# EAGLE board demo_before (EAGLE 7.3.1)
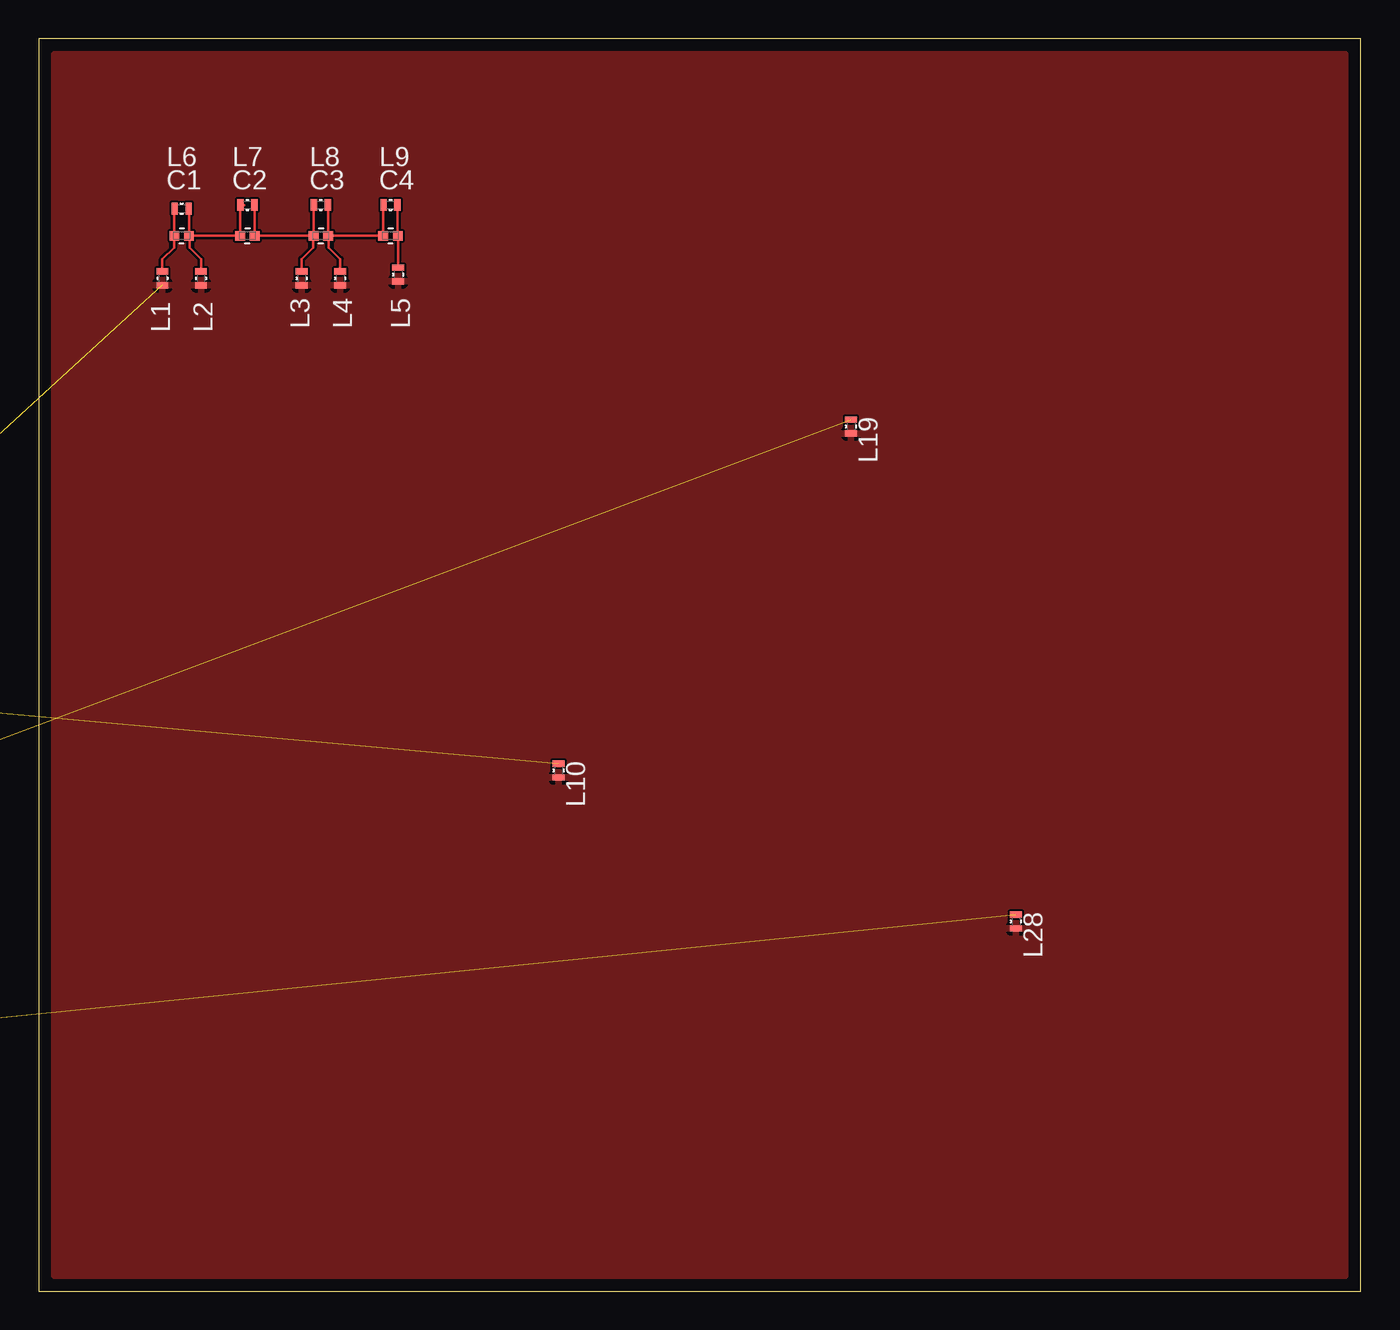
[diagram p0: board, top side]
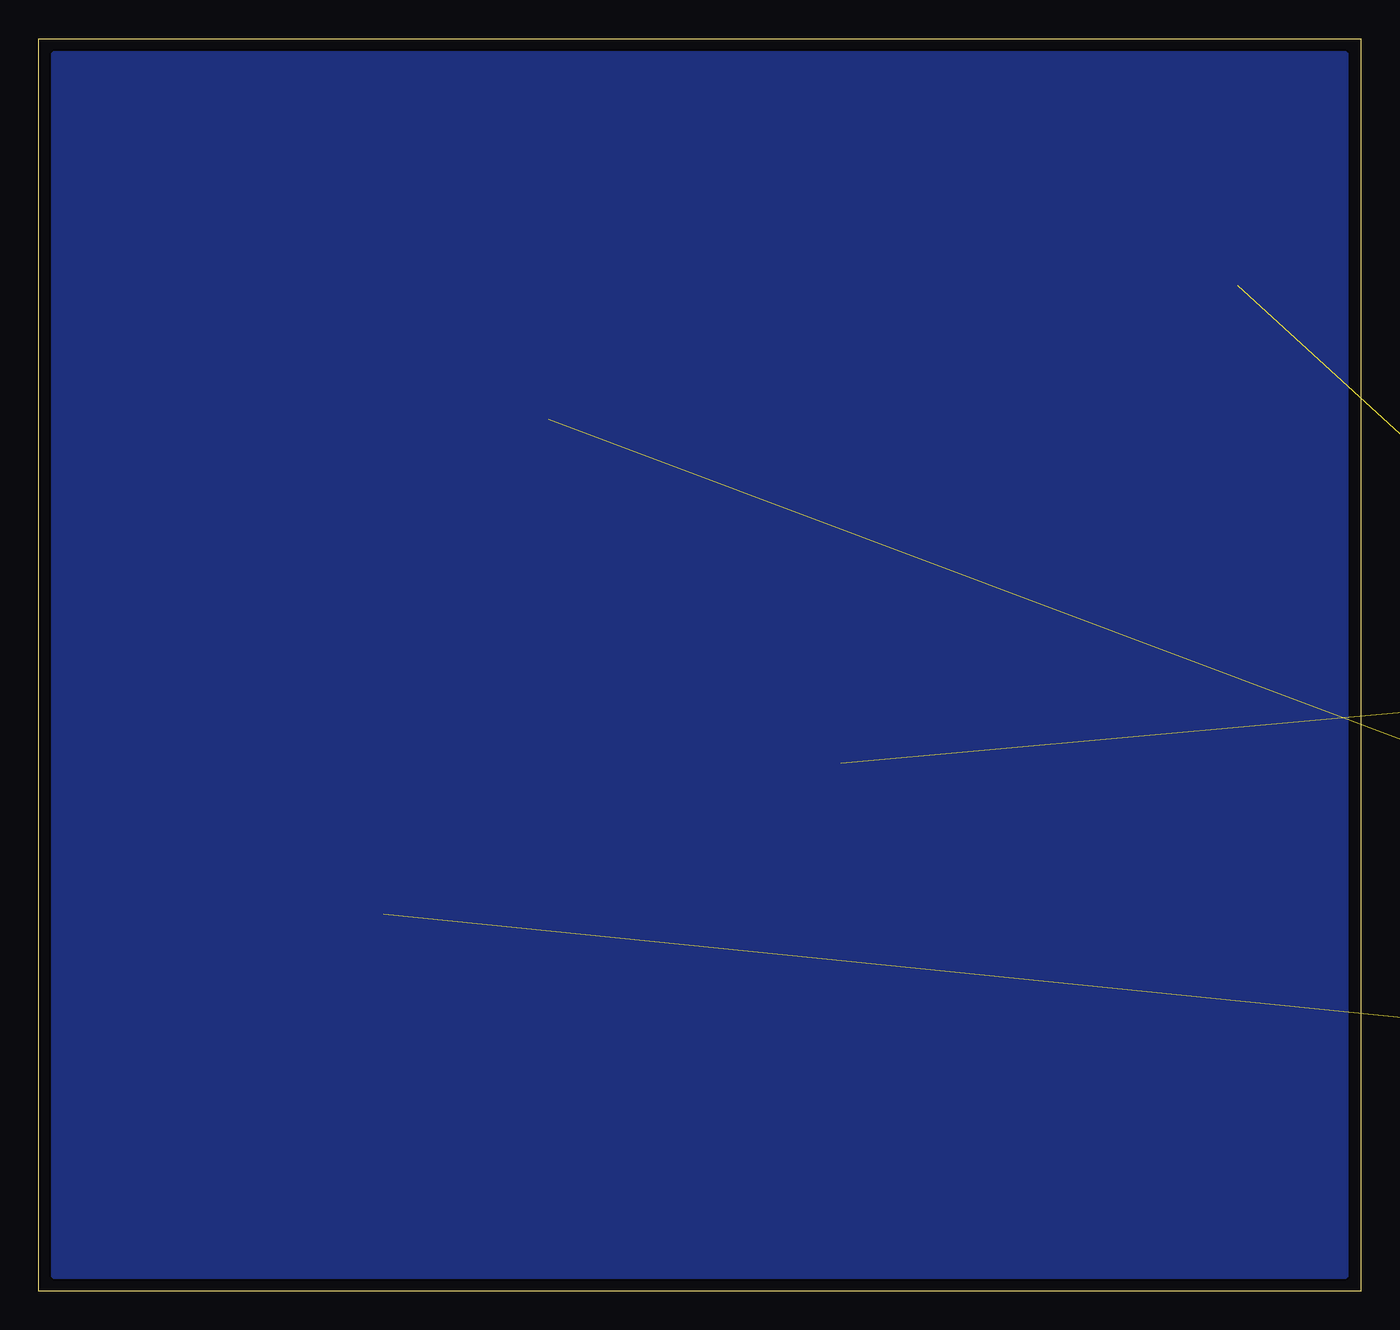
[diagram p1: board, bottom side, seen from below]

Size 85.5 x 81 mm. Coordinates in mm from the lower left corner, seen from the top.
Outline: 0,0 85.5,0 85.5,81 0,81 0,0
Copper layers (1*16): Top 0.0178mm / dielectric 59mil / Bottom 0.0178mm
Design rules "SSC-EAGLE-2Lyr_v1.0.0.3 *": minimum track width 6mil, minimum drill 14mil, track to track 6mil, track to pad 6mil, pad to pad 6mil, via to via 6mil, smd to smd 6mil, copper to edge 20mil, drill to drill 16mil, minimum pad ring 8mil, minimum via ring 8mil, stop-mask expansion 3mil, vias tented up to drill 0mil, thermal gap 10mil

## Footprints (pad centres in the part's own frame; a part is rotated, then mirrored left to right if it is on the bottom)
LTDB_PASSIVES_C0402 = smd 0.635 x 0.635: 1 -0.472,0; 2 0.472,0
LTDB_PASSIVES_R0402 = smd 0.406 x 0.762: 1 -0.447,0; 2 0.447,0

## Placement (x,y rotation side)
C1  [LTDB_PASSIVES_C0402]  9.25,68.25 0 top
C2  [LTDB_PASSIVES_C0402]  13.5,68.25 0 top
C3  [LTDB_PASSIVES_C0402]  18.25,68.25 0 top
C4  [LTDB_PASSIVES_C0402]  22.75,68.25 0 top
C5  [LTDB_PASSIVES_C0402]  not placed on the board
C6  [LTDB_PASSIVES_C0402]  not placed on the board
C7  [LTDB_PASSIVES_C0402]  not placed on the board
C8  [LTDB_PASSIVES_C0402]  not placed on the board
C9  [LTDB_PASSIVES_C0402]  not placed on the board
C10  [LTDB_PASSIVES_C0402]  not placed on the board
C11  [LTDB_PASSIVES_C0402]  not placed on the board
C12  [LTDB_PASSIVES_C0402]  not placed on the board
C13  [LTDB_PASSIVES_C0402]  not placed on the board
C14  [LTDB_PASSIVES_C0402]  not placed on the board
C15  [LTDB_PASSIVES_C0402]  not placed on the board
C16  [LTDB_PASSIVES_C0402]  not placed on the board
L1  [LTDB_PASSIVES_R0402]  8,65.5 270 top
L2  [LTDB_PASSIVES_R0402]  10.5,65.5 270 top
L3  [LTDB_PASSIVES_R0402]  17,65.5 270 top
L4  [LTDB_PASSIVES_R0402]  19.5,65.5 270 top
L5  [LTDB_PASSIVES_R0402]  23.25,65.75 270 top
L6  [LTDB_PASSIVES_R0402]  9.25,70 0 top
L7  [LTDB_PASSIVES_R0402]  13.5,70.25 0 top
L8  [LTDB_PASSIVES_R0402]  18.25,70.25 0 top
L9  [LTDB_PASSIVES_R0402]  22.75,70.25 0 top
L10  [LTDB_PASSIVES_R0402]  33.61,33.67 270 top
L11  [LTDB_PASSIVES_R0402]  not placed on the board
L12  [LTDB_PASSIVES_R0402]  not placed on the board
L13  [LTDB_PASSIVES_R0402]  not placed on the board
L14  [LTDB_PASSIVES_R0402]  not placed on the board
L15  [LTDB_PASSIVES_R0402]  not placed on the board
L16  [LTDB_PASSIVES_R0402]  not placed on the board
L17  [LTDB_PASSIVES_R0402]  not placed on the board
L18  [LTDB_PASSIVES_R0402]  not placed on the board
L19  [LTDB_PASSIVES_R0402]  52.53,55.92 270 top
L20  [LTDB_PASSIVES_R0402]  not placed on the board
L21  [LTDB_PASSIVES_R0402]  not placed on the board
L22  [LTDB_PASSIVES_R0402]  not placed on the board
L23  [LTDB_PASSIVES_R0402]  not placed on the board
L24  [LTDB_PASSIVES_R0402]  not placed on the board
L25  [LTDB_PASSIVES_R0402]  not placed on the board
L26  [LTDB_PASSIVES_R0402]  not placed on the board
L27  [LTDB_PASSIVES_R0402]  not placed on the board
L28  [LTDB_PASSIVES_R0402]  63.19,23.91 270 top
L29  [LTDB_PASSIVES_R0402]  not placed on the board
L30  [LTDB_PASSIVES_R0402]  not placed on the board
L31  [LTDB_PASSIVES_R0402]  not placed on the board
L32  [LTDB_PASSIVES_R0402]  not placed on the board
L33  [LTDB_PASSIVES_R0402]  not placed on the board
L34  [LTDB_PASSIVES_R0402]  not placed on the board
L35  [LTDB_PASSIVES_R0402]  not placed on the board
L36  [LTDB_PASSIVES_R0402]  not placed on the board

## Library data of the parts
C1-C16 L1-L36 = vnatest

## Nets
GND: L1.2 L2.2 L3.2 L4.2 L5.2 L10.2 L11.2 L12.2 L13.2 L14.2 L19.2 L20.2 L21.2 L22.2 L23.2 L28.2 L29.2 L30.2 L31.2 L32.2
IN1: C1.1 L1.1 L6.1
IN2: C5.1 L10.1 L15.1
IN3: C9.1 L19.1 L24.1
IN4: C13.1 L28.1 L33.1
N$1: C5.2 C6.1 L11.1 L15.2 L16.1
N$2: C6.2 C7.1 L12.1 L16.2 L17.1
N$3: C7.2 C8.1 L13.1 L17.2 L18.1
N$4: C9.2 C10.1 L20.1 L24.2 L25.1
N$5: C10.2 C11.1 L21.1 L25.2 L26.1
N$6: C11.2 C12.1 L22.1 L26.2 L27.1
N$7: C13.2 C14.1 L29.1 L33.2 L34.1
N$8: C14.2 C15.1 L30.1 L34.2 L35.1
N$9: C15.2 C16.1 L31.1 L35.2 L36.1
N$20: C1.2 C2.1 L2.1 L6.2 L7.1
N$21: C2.2 C3.1 L3.1 L7.2 L8.1
N$22: C3.2 C4.1 L4.1 L8.2 L9.1
OUT1: C4.2 L5.1 L9.2
OUT2: C8.2 L14.1 L18.2
OUT3: C12.2 L23.1 L27.2
OUT4: C16.2 L32.1 L36.2

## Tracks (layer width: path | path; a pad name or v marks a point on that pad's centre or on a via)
GND  (12 unrouted)
  pour Bottom: 1,80 84.5,80 84.5,1 1,1
  pour Top: 1,80 84.5,80 84.5,1 1,1
IN1
  Top 0.152: L1.1 8,66.75 8.75,67.5 8.75,68.22 C1.1 8.78,69.97 L6.1
IN2  (2 unrouted)
IN3  (2 unrouted)
IN4  (2 unrouted)
N$1  (4 unrouted)
N$2  (4 unrouted)
N$3  (4 unrouted)
N$4  (4 unrouted)
N$5  (4 unrouted)
N$6  (4 unrouted)
N$7  (4 unrouted)
N$8  (4 unrouted)
N$9  (4 unrouted)
N$20
  Top 0.152: C1.2 9.72,69.97 L6.2 | L2.1 10.5,66.75 9.75,67.5 9.75,68.22 C1.2 | 13.28,70.22 L7.1 13.03,70.22 C2.1 C1.2
N$21
  Top 0.152: L7.2 13.97,70.22 C2.2 C3.1 | C3.1 17.78,70.22 L8.1 | L3.1 17,66.75 17.75,67.5 17.75,68.22 C3.1
N$22
  Top 0.152: C3.2 C4.1 22.28,70.22 L9.1 | C3.2 18.72,70.22 L8.2 | L4.1 19.5,66.75 18.75,67.5 18.75,68.22 C3.2
OUT1
  Top 0.152: L9.2 23.22,70.22 C4.2 23.25,68.22 L5.1
OUT2  (2 unrouted)
OUT3  (2 unrouted)
OUT4  (2 unrouted)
